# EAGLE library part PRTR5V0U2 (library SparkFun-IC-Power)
A small ESD protection device. Most commonly used on USB D+/D- signals to protect large, expensive, or especially sensitive USB enabled devices.
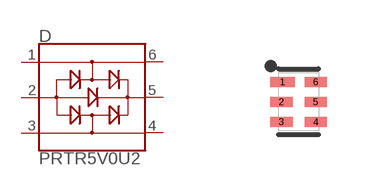
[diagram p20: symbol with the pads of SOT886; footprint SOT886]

Designator prefix D

## PRTR5V0U2F (PROD_ID: DIO-14084)  [SOT886]
1  1
2  2
3  3
4  4
5  5
6  6

## Footprint SOT886 (pad centres in mm)
SOT886 Package for "F" variant of PRTR5V0U2F
smd 0.61 x 0.25: 1 -0.405,0.5
smd 0.56 x 0.25: 2 -0.43,0; 3 -0.43,-0.5; 4 0.43,-0.5; 5 0.43,0; 6 0.43,0.5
